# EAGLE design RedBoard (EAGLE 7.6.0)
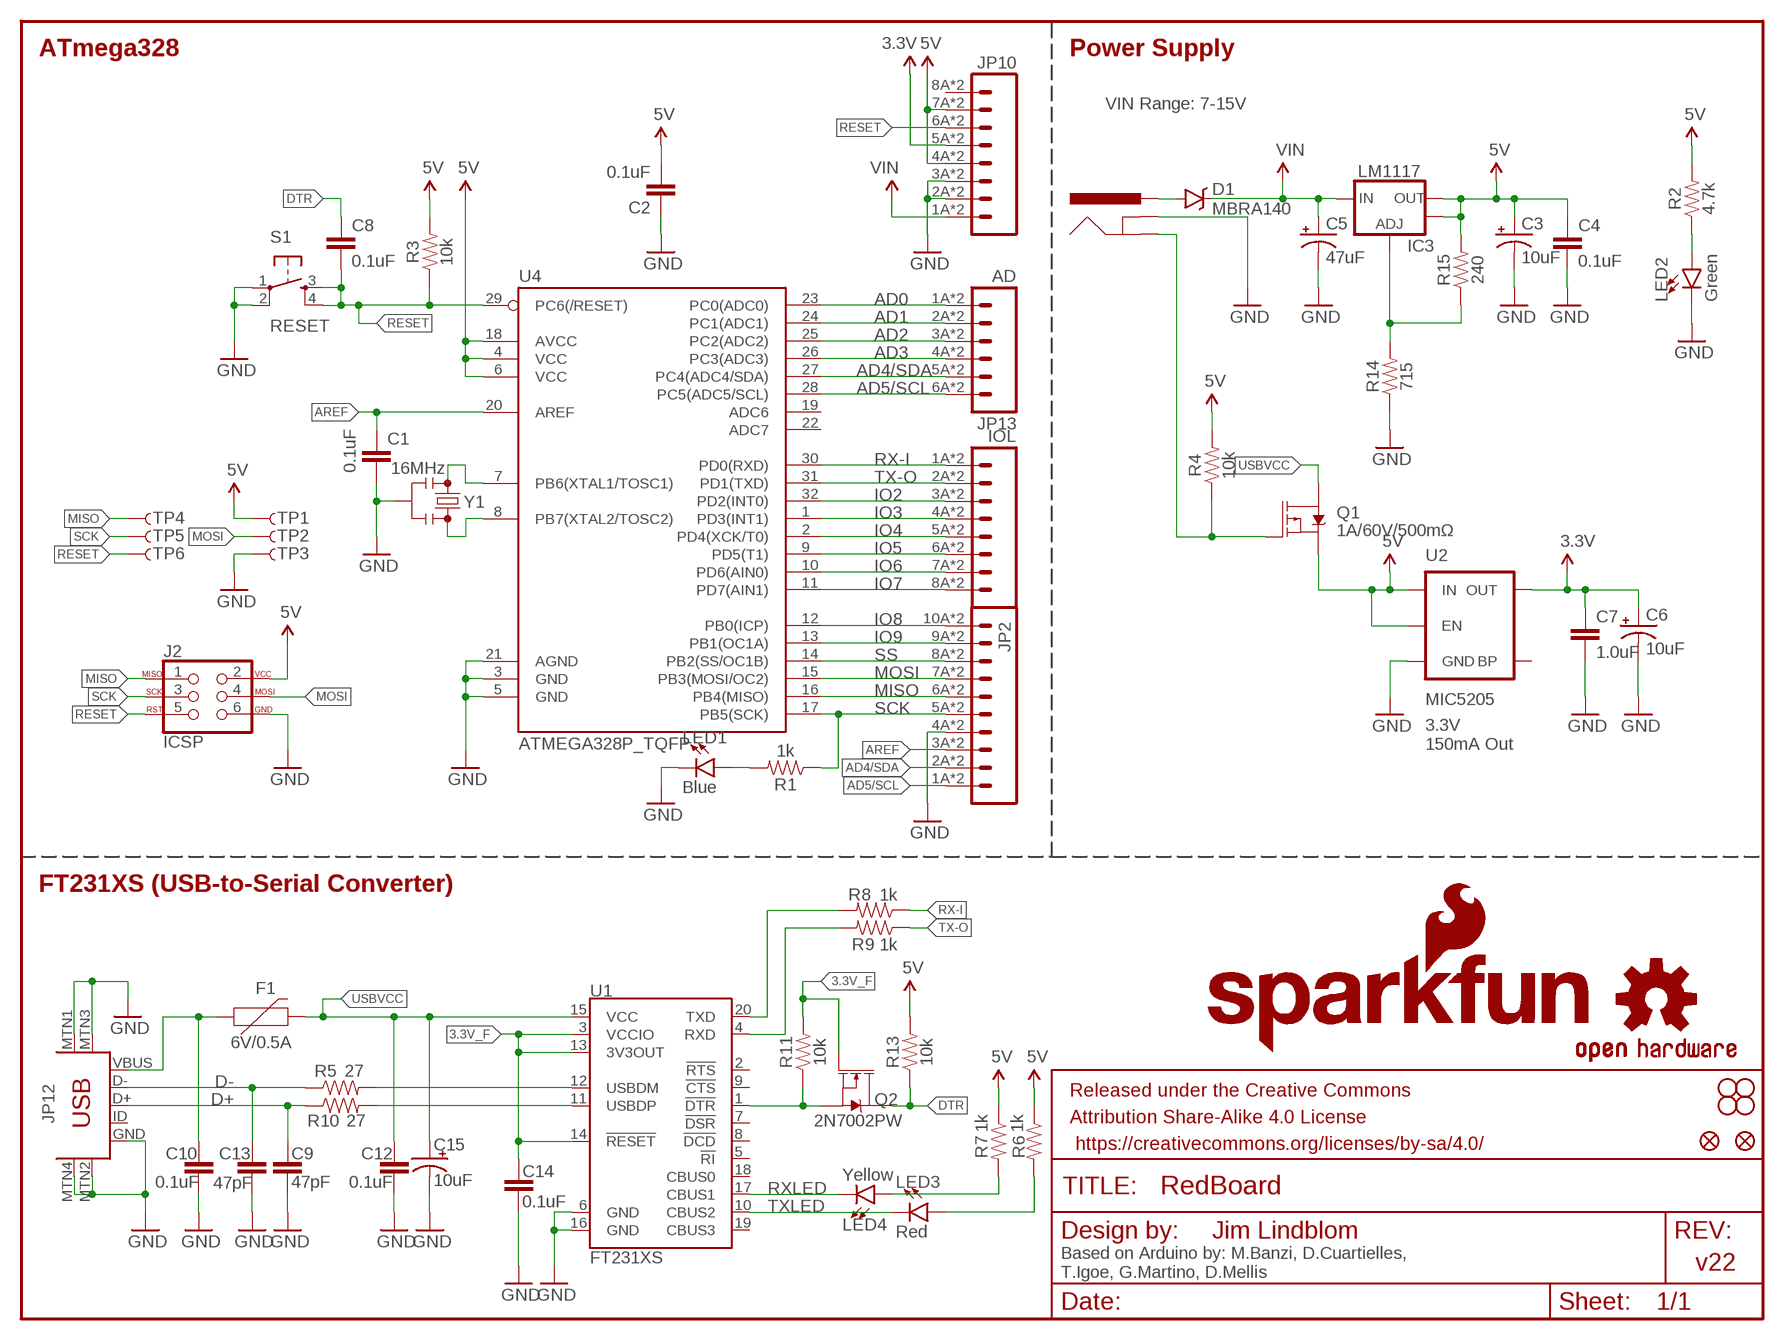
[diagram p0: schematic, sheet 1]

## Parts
C1  0.1uF  0.1UF-0603-25V-(+80/-20%)  [0603]
C2  0.1uF  0.1UF-0603-25V-(+80/-20%)  [0603]
C3  10uF  10UF-POLAR-EIA3216-16V-10%(TANT)  [EIA3216]
C4  0.1uF  0.1UF-0603-25V-(+80/-20%)  [0603]
C5  47uF  47UF-POLAR-PANASONIC_D-35V-20%  [PANASONIC_D]
C6  10uF  10UF-POLAR-EIA3216-16V-10%(TANT)  [EIA3216]
C7  1.0uF  1.0UF-0603-16V-10%  [0603]
C8  0.1uF  0.1UF-0603-25V-(+80/-20%)  [0603]
C9  47pF  47PF-0603-50V-5%  [0603]
C10  0.1uF  0.1UF-0603-25V-(+80/-20%)  [0603]
C12  0.1uF  0.1UF-0603-25V-(+80/-20%)  [0603]
C13  47pF  47PF-0603-50V-5%  [0603]
C14  0.1uF  0.1UF-0603-25V-(+80/-20%)  [0603]
C15  10uF  10UF-POLAR-EIA3216-16V-10%(TANT)  [EIA3216]
D1  MBRA140  [SMA-DIODE]
F1  6V/0.5A  PTC-HALF_AMP  [1206]
FRAME2  FRAME-LETTER  [CREATIVE_COMMONS]
IC3  LM1117  V_REG_LM1117ALT1  [SOT223-ALT1]
J2  ICSP  AVR_SPI_PROG_3X2SMD  [2X3_SMT_POSTS]
J3  POWER_JACKSUPER_BOMB_DIGITY  [POWER_JACK_SMD_OVERPASTE_SUPER_BOMB_DIGITY]
JP1  SFE_LOGO_NAME.1_INCH  [SFE_LOGO_NAME_.1]
JP2  M10SMD_COMBO  [1X10_SMD_COMBINED]
JP3  STAND-OFF  [STAND-OFF]
JP4  STAND-OFF  [STAND-OFF]
JP5  STAND-OFF  [STAND-OFF]
JP6  STAND-OFF  [STAND-OFF]
JP7  SFE_LOGO_FLAME.1_INCH  [SFE_LOGO_FLAME_.1]
JP8  FIDUCIAL1X2  [FIDUCIAL-1X2]
JP9  FIDUCIAL1X2  [FIDUCIAL-1X2]
JP10  M08SMD-COMBO  [1X08_SMD_COMBINED]
JP11  IOL  M08SMD-COMBO  [1X08_SMD_COMBINED]
JP12  USB-MINIB-5PIN  [USB-MINIB]
JP13  AD  M06SMD-STRAIGHT-COMBO  [1X06_SMD_STRAIGHT_COMBO]
LED1  Blue  LED1206  [LED-1206]
LED2  Green  LED1206  [LED-1206]
LED3  Red  LED1206  [LED-1206]
LED4  Yellow  LED1206  [LED-1206]
Q1  1A/60V/500mΩ  MOSFET-PCH-ZXMP6A13F  [SOT23-3]
Q2  2N7002PW  MOSFET-NCH-2N7002PW  [SOT323]
R1  1k  1KOHM-0603-1/10W-1%  [0603]
R2  4.7k  4.7KOHM-0603-1/10W-1%  [0603]
R3  10k  10KOHM-0603-1/10W-1%  [0603]
R4  10k  10KOHM-0603-1/10W-1%  [0603]
R5  27  27OHM-0603-1/10W-1%  [0603]
R6  1k  1KOHM-0603-1/10W-1%  [0603]
R7  1k  1KOHM-0603-1/10W-1%  [0603]
R8  1k  1KOHM-0603-1/10W-1%  [0603]
R9  1k  1KOHM-0603-1/10W-1%  [0603]
R10  27  27OHM-0603-1/10W-1%  [0603]
R11  10k  10KOHM-0603-1/10W-1%  [0603]
R13  10k  10KOHM-0603-1/10W-1%  [0603]
R14  715  715OHM-0603-1/10W-1%  [0603]
R15  240  240OHM-0603-1/10W-1%  [0603]
S1  RESET  SWITCH_SPST_4_PINSQUARE  [TACTILE-SWITCH-SMD]
TP1  TP-3x5  TEST-POINT3X5  [PAD.03X.05]
TP2  TP-3x5  TEST-POINT3X5  [PAD.03X.05]
TP3  TP-3x5  TEST-POINT3X5  [PAD.03X.05]
TP4  TP-3x5  TEST-POINT3X5  [PAD.03X.05]
TP5  TP-3x5  TEST-POINT3X5  [PAD.03X.05]
TP6  TP-3x5  TEST-POINT3X5  [PAD.03X.05]
U1  FT231XS  [SSOP20_L]
U2  MIC5205  MIC52053.3V  [SOT23-5]
U4  ATMEGA328P_TQFP  [TQFP32-08]
U$16  OSHW-LOGOS  [OSHW-LOGO-S]
Y1  16MHz  RESONATOR-16MHZSMD_3.2X1.3  [RESONATOR-SMD-3.2X1.3]

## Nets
3.3V: C6.+ C7.1 JP10.5A JP10.5B U2.5(OUT)
3.3V_F: C14.1 Q2.1(G) R11.2 U1.3(VCCIO) U1.13(3V3OUT) U1.14(!RESET)
5V: C2.2 C3.+ C4.1 IC3.2(OUT) IC3.4(OUT) J2.2 JP10.4A JP10.4B JP10.7A JP10.7B Q1.2(S) R2.2 R3.2 R4.2 R6.1 R7.1 R13.2 R15.2 TP1.P$1 U2.1(IN) U2.3(EN) U4.4(VCC) U4.6(VCC) U4.18(AVCC)
AD0: JP13.1A JP13.1B U4.23(PC0(ADC0))
AD1: JP13.2A JP13.2B U4.24(PC1(ADC1))
AD2: JP13.3A JP13.3B U4.25(PC2(ADC2))
AD3: JP13.4A JP13.4B U4.26(PC3(ADC3))
AD4/SDA: JP2.2A JP2.2B JP13.5A JP13.5B U4.27(PC4(ADC4/SDA))
AD5/SCL: JP2.1A JP2.1B JP13.6A JP13.6B U4.28(PC5(ADC5/SCL))
AREF: C1.1 JP2.3A JP2.3B U4.20(AREF)
D+: C9.1 JP12.D+ R10.1
D-: C13.1 JP12.D- R5.1
DTR: C8.1 Q2.3(D) R13.1
FTDI_DTR: Q2.2(S) R11.1 U1.1(!DTR)
GND: C1.2 C2.1 C3.- C4.2 C5.- C6.- C7.2 C9.2 C10.2 C12.2 C13.2 C14.2 C15.- J2.6 J3.GND(GNDBREAK) JP2.4A JP2.4B JP10.2A JP10.2B JP10.3A JP10.3B JP12.GND JP12.MTN1(MTN2) JP12.MTN2(MTN3) JP12.MTN3(MTN1) JP12.MTN4 LED1.C LED2.C R14.1 S1.1 S1.2 TP3.P$1 U1.6(GND) U1.16(GND) U2.2(GND) U4.3(GND) U4.5(GND) U4.21(AGND) Y1.2
INSERT: J3.P$4(GND) Q1.1(G) R4.1
IO2: JP11.3A JP11.3B U4.32(PD2(INT0))
IO3: JP11.4A JP11.4B U4.1(PD3(INT1))
IO4: JP11.5A JP11.5B U4.2(PD4(XCK/T0))
IO5: JP11.6A JP11.6B U4.9(PD5(T1))
IO6: JP11.7A JP11.7B U4.10(PD6(AIN0))
IO7: JP11.8A JP11.8B U4.11(PD7(AIN1))
IO8: JP2.10A JP2.10B U4.12(PB0(ICP))
IO9: JP2.9A JP2.9B U4.13(PB1(OC1A))
MISO: J2.1 JP2.6A JP2.6B TP4.P$1 U4.16(PB4(MISO))
MOSI: J2.4 JP2.7A JP2.7B TP2.P$1 U4.15(PB3(MOSI/OC2))
N$1: LED1.A R1.2
N$2: LED2.A R2.1
N$3: U4.7(PB6(XTAL1/TOSC1)) Y1.1
N$4: U4.8(PB7(XTAL2/TOSC2)) Y1.3
N$6: R5.2 U1.12(USBDM)
N$7: R10.2 U1.11(USBDP)
N$8: LED3.A R6.2
N$10: LED4.A R7.2
N$15: IC3.1(ADJ) R14.2 R15.1
PWRIN: D1.A J3.VIN0(PWR)
RESET: C8.2 J2.5 JP10.6A JP10.6B R3.1 S1.3 S1.4 TP6.P$1 U4.29(PC6(/RESET))
RX-I: JP11.1A JP11.1B R8.1 U4.30(PD0(RXD))
RXD: R9.2 U1.4(RXD)
RXLED: LED4.C U1.17(CBUS1)
SCK: J2.3 JP2.5A JP2.5B R1.1 TP5.P$1 U4.17(PB5(SCK))
SS: JP2.8A JP2.8B U4.14(PB2(SS/OC1B))
TX-O: JP11.2A JP11.2B R9.1 U4.31(PD1(TXD))
TXD: R8.2 U1.20(TXD)
TXLED: LED3.C U1.10(CBUS2)
USBVCC: C12.1 C15.+ F1.2 Q1.3(D) U1.15(VCC)
VIN: C5.+ D1.C IC3.3(IN) JP10.1A JP10.1B
VUSB: C10.1 F1.1 JP12.VBUS
Unconnected: JP10.8A JP10.8B JP12.ID U1.2(!RTS) U1.5(!RI) U1.7(!DSR) U1.8(!DCD) U1.9(!CTS) U1.18(CBUS0) U1.19(CBUS3) U2.4(BP) U4.19(ADC6) U4.22(ADC7)

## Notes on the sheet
- ATmega328 | Power Supply
- VIN Range: 7-15V
- 3.3V
  150mA Out
- FT231XS (USB-to-Serial Converter)
- Jim Lindblom
- v22
- Based on Arduino by: M.Banzi, D.Cuartielles, 
  T.Igoe, G.Martino, D.Mellis

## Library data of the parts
C1 C2 C4 C8 C10 C12 C14 = SparkFun-Capacitors:0.1UF: 0.1µF ceramic capacitors; PROD_ID: CAP-00810
C3 C6 C15 = SparkFun-Capacitors:10UF-POLAR: 10.0µF polarized capacitors; PROD_ID: CAP-00811
C5 = SparkFun-Capacitors:47UF-POLAR: 47µF polarized capacitors; PROD_ID: CAP-08478
C7 = SparkFun-Capacitors:1.0UF: 1µF ceramic capacitors; PROD_ID: CAP-00868
C9 C13 = SparkFun-Capacitors:47PF: 47pF ceramic capacitors; PROD_ID: CAP-08913
D1 = SparkFun-DiscreteSemi:MBRA140: 40V, 1A Schottky rectifier; PROD_ID: DIO-08053
F1 = SparkFun-Fuses:PTC: Resettable Fuse PTC; PROD_ID: RES-08585
FRAME2 = SparkFun-Aesthetics:FRAME-LETTER: Schematic Frame
IC3 = Testing:V_REG_LM1117: Voltage Regulator LM1117 Standard adjustable voltage regulator but in SMD form. Spark Fun Electronics SKU : COM-00595; PROD_ID: VREG-08170
J2 = SparkFun-Connectors:AVR_SPI_PROG_3X2: AVR ISP 6 Pin This is the reduced ISP connector for AVR programming. Common on Arduino. This footprint will take up less PCB space and can be used with a 10-pin to 6-pin adapter such as SKU: BOB-08508 **Special note about "TEST_POINT" package. The stop mask is on the top side, so if you want your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; PROD_ID: CONN-11415
J3 = Testing:POWER_JACK: Power Jack This is the standard 5.5mm barrel jack for power. The PTH is the most common, proven, reliable, footprint. All others are experimental. The Slot footprint only works if the mill layer is transmitted to the PCB fab house so be warned. Spark Fun Electronics SKU : PRT-00119. Mating wall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; PROD_ID: CONN-08106
JP1 = SparkFun-Aesthetics:SFE_LOGO_NAME: SFE Logo, name only
JP2 = SparkFun-Connectors:M10: Header 10 Standard 10-pin 0.1" header. Use with straight break away headers (SKU : PRT-00116), right angle break away headers (PRT-00553), swiss pins (PRT-00743), machine pins (PRT-00117), and female headers (PRT-00115).; PROD_ID: CONN-11219
JP3-JP6 = SparkFun:STAND-OFF: Stand Off
JP7 = SparkFun-Aesthetics:SFE_LOGO_FLAME: SFE Logo, flame only
JP8 JP9 = SparkFun:FIDUCIAL: Fiducial Alignment Points
JP10 JP11 = SparkFun-Connectors:M08: Header 8 Standard 8-pin 0.1" header. Use with straight break away headers (SKU : PRT-00116), right angle break away headers (PRT-00553), swiss pins (PRT-00743), machine pins (PRT-00117), and female headers (PRT-00115).; PROD_ID: CONN-10204
JP12 = SparkFun-Connectors:USB-MINIB: Mini-USB "B" connector with 5th pin broken out. Created new symbol breaking out 5th "ID" pin in mini/micro USB connector spec. See: http://en.wikipedia.org/wiki/Mini_usb#Cables. Uses same footprint as 4-pin symbol. Also added pins to connect to mounting / shield pads if required (probably not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; PROD_ID: CONN-08193
JP13 = SparkFun-Connectors:M06: Header 6 Standard 6-pin 0.1" header. Use with straight break away headers (SKU : PRT-00116), right angle break away headers (PRT-00553), swiss pins (PRT-00743), machine pins (PRT-00117), and female headers (PRT-00115). Molex polarized connector foot print use with SKU : PRT-08094 with associated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; PROD_ID: CONN-10203
LED1 = SparkFun-LED:LED: LED (Generic); PROD_ID: DIO-09911
LED2 = SparkFun-LED:LED: LED (Generic); PROD_ID: DIO-09910
LED3 = SparkFun-LED:LED: LED (Generic); PROD_ID: DIO-09912
LED4 = SparkFun-LED:LED: LED (Generic); PROD_ID: DIO-09909
Q1 = SparkFun-DiscreteSemi:MOSFET-PCH: P-channel MOSFETs Voltage controlled devices that allow control of high current outputs.; PROD_ID: TRANS-08285
Q2 = SparkFun-DiscreteSemi:MOSFET-NCH: N-channel MOSFETs Voltage controlled devices that allow control of high current outputs.; PROD_ID: TRANS-11151; VALUE: 310mA/60V/1.6Ω
R1 R6-R9 = SparkFun-Resistors:1KOHM: 1kΩ resistor; PROD_ID: RES-07856
R2 = SparkFun-Resistors:4.7KOHM: 4.7kΩ resistor; PROD_ID: RES-07857
R3 R4 R11 R13 = SparkFun-Resistors:10KOHM: 10kΩ resistor; PROD_ID: RES-00824
R5 R10 = SparkFun-Resistors:27OHM: 27Ω resistor; PROD_ID: RES-09334
R14 = SparkFun-Resistors:715OHM: 715Ω resistor; PROD_ID: RES-07850
R15 = SparkFun-Resistors:240OHM: 240Ω resistor; PROD_ID: RES-07849
S1 = SparkFun-Electromechanical:SWITCH_SPST_4_PIN; PROD_ID: SWCH-08247
TP1-TP4 TP6 = SparkFun-Connectors:TEST-POINT: Bare copper test points for troubleshooting or ICT
TP5 = SparkFun-Passives:TEST-POINT: Bare copper test points for troubleshooting or ICT
U1 = SparkFun-IC-Comms:FT231X: FTDI FT231X Full Speed USB to Full-handshake UART This USB2.0 Full Speed IC offers a compact bridge to full handshake UART interfaces. The device is a UART, capable of operating up to 3MBaud, with low power consumption (8mA). The FT231X includes the complete FT-X series feature set and enables USB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; PROD_ID: IC-11524
U2 = SparkFun-PowerIC:MIC5205: MIC5205 150mA vreg 3.3V - VREG-00822 5V - VREG-00823; PROD_ID: VREG-00822
U4 = SparkFun-IC-Microcontroller:ATMEGA328P_TQFP; PROD_ID: IC-09069
U$16 = SparkFun-Aesthetics:OSHW-LOGO: Open Source Hardware Logo
Y1 = SparkFun-Clocks:RESONATOR-16MHZ: 16MHz Resonator Digikey Example Frequency: 16MHz Frequency Stability: &plusmn;0.3% Frequency Tolerance: &plusmn;0.5% Capacitance: 15pF; PROD_ID: XTAL-08900

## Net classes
0 default: width 0.152 mm, drill 0.305 mm, clearance 0.152 mm

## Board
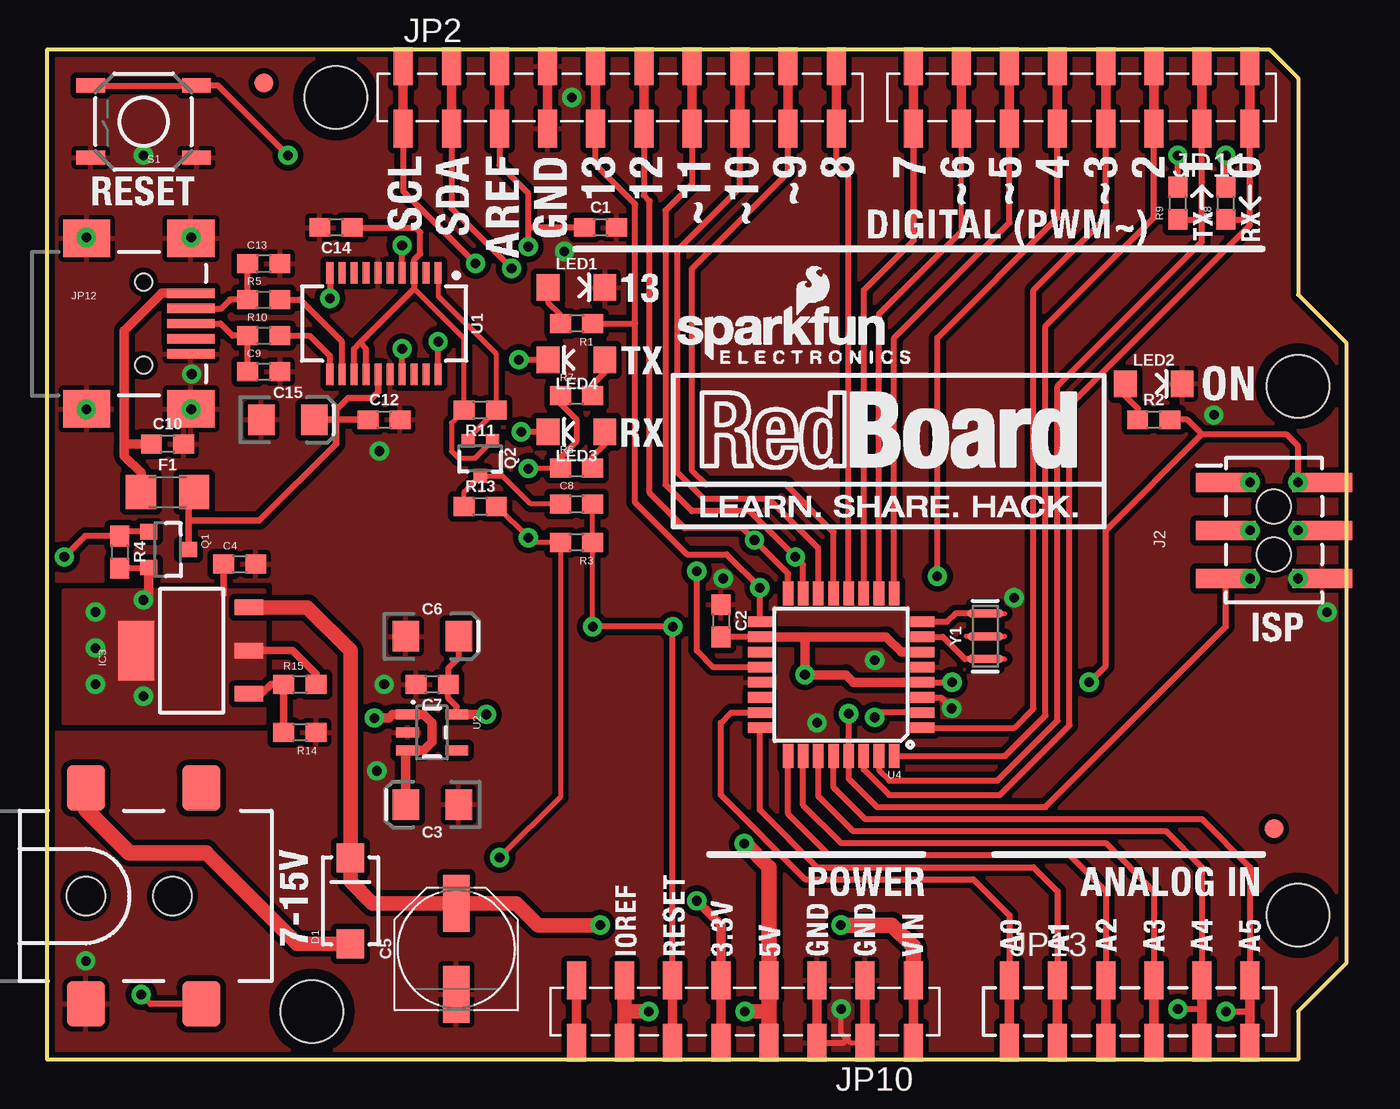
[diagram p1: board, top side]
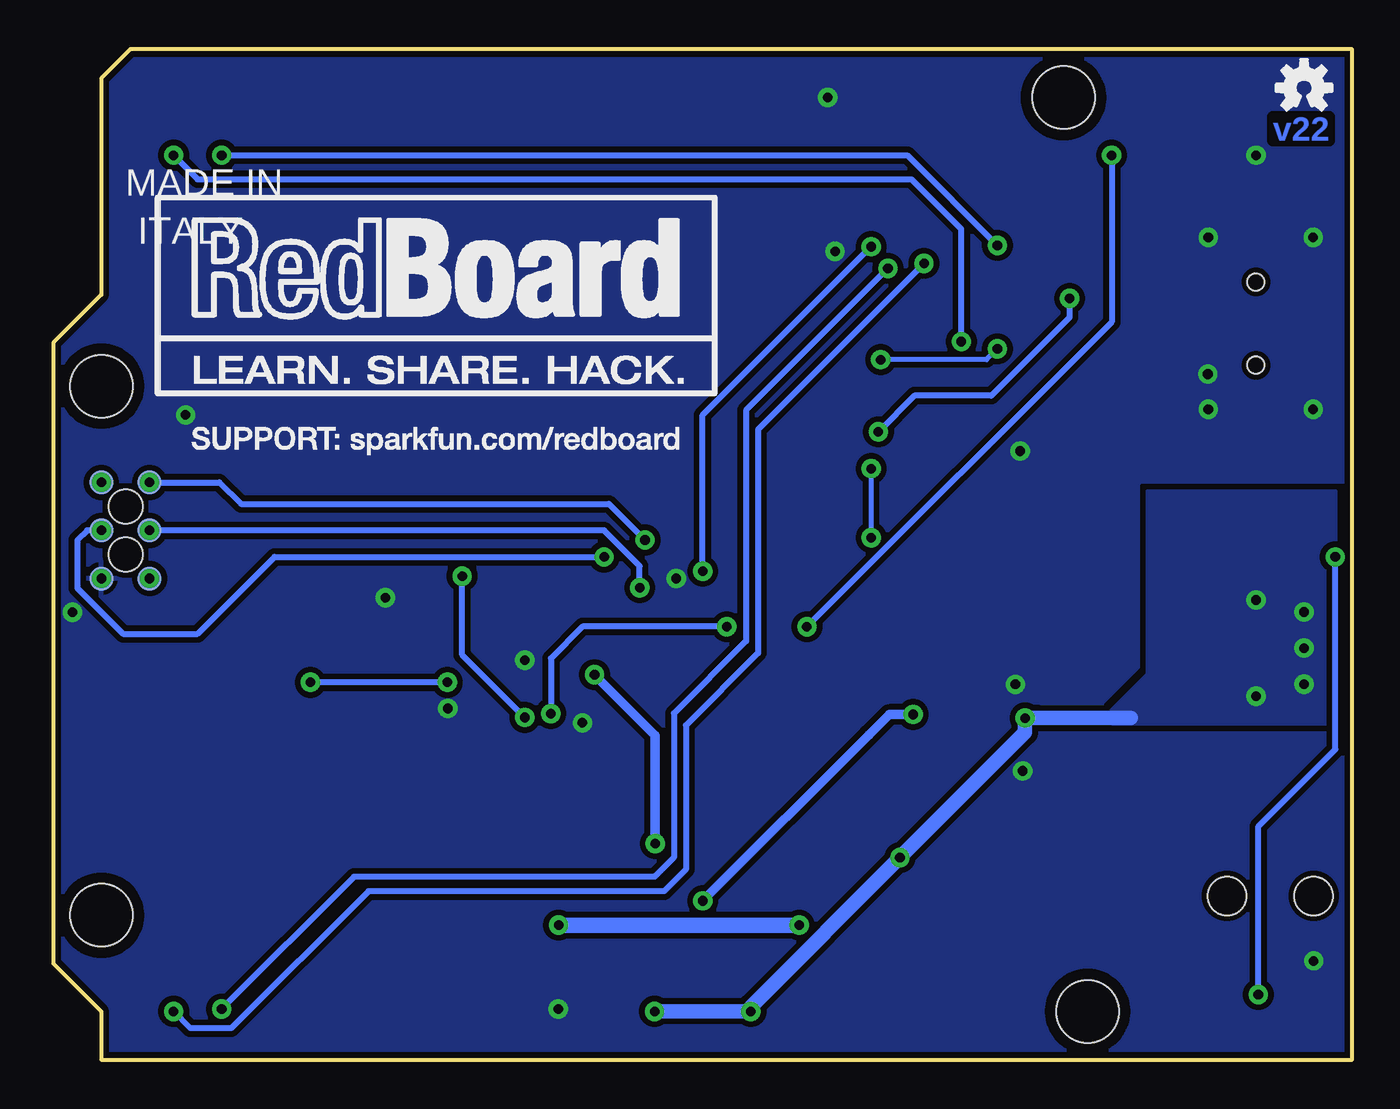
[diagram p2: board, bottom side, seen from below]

Size 68.58 x 53.34 mm. Coordinates in mm from the lower left corner, seen from the top.
Outline: 0,53.34 64.52,53.34 66.04,51.82 66.04,40.39 68.58,37.85 68.58,5.08 66.04,2.54 66.04,0 0,0 0,53.34
Copper layers (1*16): Top 0.035mm / dielectric 1.5mm / Bottom 0.035mm
Design rules "SparkFun-2-layer": minimum track width 7mil, minimum drill 15mil, track to track 8mil, track to pad 8mil, pad to pad 8mil, via to via 8mil, smd to smd 8mil, copper to edge 8mil, drill to drill 8mil, minimum pad ring 12mil, minimum via ring 10mil, stop-mask expansion 4mil, vias tented up to drill 20mil, thermal gap 10mil
vRestrict: area 0.6,22.4 to 2,30.6; area 5.7,23.1 to 7.4,30.6; area 47.9,10.8 to 48.5,11.3; area 50.4,10.7 to 50.9,11.6; area 11.3,29.3 to 12.7,31.6; area 0.3,13 to 9.4,25

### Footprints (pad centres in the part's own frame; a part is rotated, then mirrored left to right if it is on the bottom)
0603 = smd 1.1 x 1: 1 -0.85,0; 2 0.85,0
EIA3216 = smd 1.4 x 1.6: + 1.4,0; - -1.4,0
PANASONIC_D = smd 3 x 1.4: + 2.4,0; - -2.4,0
SMA-DIODE = smd 1.524 x 1.47: A -2.277,0; C 2.277,0
1206 = smd 1.6 x 1.8: 1 -1.4,0; 2 1.4,0
SOT223-ALT1 = smd 0.813 x 1.524: 1 -2.271,-3.02; 2 0,-3.02; 3 2.288,-3.02 | smd 3.124 x 1.905: 4 0,2.921
2X3_SMT_POSTS = smd 1 x 3.17: 1 -2.54,-2.54; 2 -2.54,2.54; 3 0,-2.54; 4 0,2.54; 5 2.54,-2.54; 6 2.54,2.54 | hole 1.8: -1.27,0; 1.27,0
POWER_JACK_SMD_OVERPASTE_SUPER_BOMB_DIGITY = smd 2 x 2.4: GND 0,-5.7; P$4 6.1,-5.7; VIN0 0,5.7; VIN1 6.1,5.7 | hole 2.032: 0,0; 4.572,0
1X10_SMD_COMBINED = smd 1 x 2: 1A 0,1.65; 1B 0,-1.65; 2A 2.54,1.65; 2B 2.54,-1.65; 3A 5.08,1.65; 3B 5.08,-1.65; 4A 7.62,1.65; 4B 7.62,-1.65; 5A 10.16,1.65; 5B 10.16,-1.65; 6A 12.7,1.65; 6B 12.7,-1.65; 7A 15.24,1.65; 7B 15.24,-1.65; 8A 17.78,1.65; 8B 17.78,-1.65; 9A 20.32,1.65; 9B 20.32,-1.65; 10A 22.86,1.65; 10B 22.86,-1.65
STAND-OFF = hole 3.302: 0,0
FIDUCIAL-1X2 = smd 1 x 1: 1 0,0
1X08_SMD_COMBINED = smd 1 x 2: 1A 0,1.65; 1B 0,-1.65; 2A 2.54,-1.65; 2B 2.54,1.65; 3A 5.08,1.65; 3B 5.08,-1.65; 4A 7.62,-1.65; 4B 7.62,1.65; 5A 10.16,1.65; 5B 10.16,-1.65; 6A 12.7,-1.65; 6B 12.7,1.65; 7A 15.24,1.65; 7B 15.24,-1.65; 8A 17.78,-1.65; 8B 17.78,1.65
USB-MINIB = smd 2.5 x 0.5: D+ 2.5,0; D- 2.5,0.8; GND 2.5,-1.6; ID 2.5,-0.8; VBUS 2.5,1.6 | smd 2.5 x 2: MTN1 -3,4.5; MTN2 2.5,4.5; MTN3 -3,-4.5; MTN4 2.5,-4.5 | hole 0.9: 0,2.2; 0,-2.2
1X06_SMD_STRAIGHT_COMBO = smd 1 x 2: 1A 0,-1.65; 1B 0,1.65; 2A 2.54,1.65; 2B 2.54,-1.65; 3A 5.08,-1.65; 3B 5.08,1.65; 4A 7.62,1.65; 4B 7.62,-1.65; 5A 10.16,-1.65; 5B 10.16,1.65; 6A 12.7,1.65; 6B 12.7,-1.65
LED-1206 = smd 1.2 x 1.4: A -1.5,0; C 1.5,0
SOT23-3 = smd 0.8 x 0.9: 1 -0.95,-1; 2 0.95,-1; 3 0,1.1
SOT323 = smd 0.7 x 0.7: 1 -0.65,-0.925; 2 0.65,-0.925; 3 0,0.925
TACTILE-SWITCH-SMD = smd 1.524 x 0.762: 1 -2.794,1.905; 2 2.794,1.905; 3 -2.794,-1.905; 4 2.794,-1.905
PAD.03X.05 = smd 1.27 x 1.27: P$1 0,0
SSOP20_L = smd 0.381 x 1.143: 1 -2.857,-2.68; 2 -2.223,-2.68; 3 -1.587,-2.68; 4 -0.953,-2.68; 5 -0.318,-2.68; 6 0.318,-2.68; 7 0.953,-2.68; 8 1.587,-2.68; 9 2.223,-2.68; 10 2.857,-2.68; 11 2.857,2.68; 12 2.223,2.68; 13 1.587,2.68; 14 0.953,2.68; 15 0.318,2.68; 16 -0.318,2.68; 17 -0.953,2.68; 18 -1.587,2.68; 19 -2.223,2.68; 20 -2.857,2.68
SOT23-5 = smd 0.55 x 1.2: 1 -0.95,-1.3; 2 0,-1.3; 3 0.95,-1.3; 4 0.95,1.3; 5 -0.95,1.3
TQFP32-08 = smd 1.27 x 0.559: 1 -4.293,2.8; 2 -4.293,2; 3 -4.293,1.2; 4 -4.293,0.4; 5 -4.293,-0.4; 6 -4.293,-1.2; 7 -4.293,-2; 8 -4.293,-2.8; 17 4.293,-2.8; 18 4.293,-2; 19 4.293,-1.2; 20 4.293,-0.4; 21 4.293,0.4; 22 4.293,1.2; 23 4.293,2; 24 4.293,2.8 | smd 0.559 x 1.27: 9 -2.8,-4.293; 10 -2,-4.293; 11 -1.2,-4.293; 12 -0.4,-4.293; 13 0.4,-4.293; 14 1.2,-4.293; 15 2,-4.293; 16 2.8,-4.293; 25 2.8,4.293; 26 2,4.293; 27 1.2,4.293; 28 0.4,4.293; 29 -0.4,4.293; 30 -1.2,4.293; 31 -2,4.293; 32 -2.8,4.293
RESONATOR-SMD-3.2X1.3 = smd 0.45 x 1.905: 1 -1.2,0; 2 0,0; 3 1.2,0

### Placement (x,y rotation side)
C1  29.21,43.94 0 top
C2  35.56,23.17 270 top
C3  20.32,13.46 180 top
C4  10.16,26.16 0 top
C5  21.59,5.84 90 top
C6  20.32,22.35 0 top
C7  20.32,19.81 180 top
C8  27.94,29.34 0 top
C9  11.43,36.32 0 top
C10  6.35,32.51 0 top
C12  17.78,33.78 0 top
C13  11.43,42.04 0 top
C14  15.24,43.94 180 top
C15  12.7,33.78 0 top
D1  16,8.38 90 top
F1  6.35,29.97 0 top
FRAME2  not placed on the board
IC3  7.62,21.59 90 top
J2  64.77,27.94 270 top
J3  2.03,8.64 0 top
JP1  32.79,36.45 0 top
JP2  18.8,50.8 0 top
JP3  13.97,2.54 0 top
JP4  66.04,7.62 0 top
JP5  66.04,35.56 0 top
JP6  15.24,50.8 0 top
JP7  39.27,38.99 0 top
JP8  64.77,12.19 0 top
JP9  11.43,51.56 0 top
JP10  45.72,2.54 180 top
JP11  63.5,50.8 180 top
JP12  5.08,38.86 0 top
JP13  50.8,2.54 0 top
LED1  27.94,40.77 0 top
LED2  58.42,35.69 0 top
LED3  27.94,33.15 180 top
LED4  27.94,36.96 180 top
Q1  6.35,26.92 270 top
Q2  22.86,31.75 180 top
R1  27.94,38.86 180 top
R2  58.42,33.78 0 top
R3  27.94,27.3 180 top
R4  3.81,26.8 270 top
R5  11.43,40.13 0 top
R6  27.94,31.24 0 top
R7  27.94,35.05 0 top
R8  62.23,45.21 90 top
R9  59.69,45.21 90 top
R10  11.43,38.23 0 top
R11  22.86,34.29 180 top
R13  22.86,29.21 0 top
R14  13.34,17.27 180 top
R15  13.34,19.81 0 top
S1  5.08,49.53 180 top
TP1  66.04,30.48 0 bottom
TP2  66.04,27.94 0 bottom
TP3  66.04,25.4 0 bottom
TP4  63.5,30.48 0 bottom
TP5  63.5,27.94 0 bottom
TP6  63.5,25.4 0 bottom
U1  17.78,38.86 180 top
U2  20.32,17.27 270 top
U4  41.91,20.32 180 top
U$16  2.54,51.31 0 bottom
Y1  49.53,22.35 90 top

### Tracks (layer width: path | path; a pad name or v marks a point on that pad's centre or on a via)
3.3V  (via drill 0.51)
  Top 0.305: U2.5 21.62,18.64 21.17,19.09 C7.1 21.17,20.66 21.72,21.21 C6.+
  Top 0.508: JP10.5A 35.56,7.11 v34.29,8.38 | U2.5 v23.18,18.22
  Bottom 0.508: v34.29,8.38 25.53,17.14 25.52,17.14 24.45,18.22 v23.18,18.22
3.3V_F
  Top 0.254: 19.37,40.7 22.01,38.06 R11.2 21.34,33.62 21.34,32.13 21.72,31.75 22.59,31.75 Q2.1
  Top 0.305: C14.1 19.43,43.94 19.68,43.69 19.68,42.55 19.37,42.23 U1.3 19.37,40.7 16.51,37.85 | U1.13 16.19,37.53 16.51,37.85 | U1.14 16.83,37.53 16.51,37.85
5V  (via drill 0.51, 0.51 pad 0.51)
  Top 0.254: 27.09,31.2 v25.4,31.2 | R13.2 23.75,29.21 v25.4,27.56 25.65,27.3 R3.2 27.09,13.88 v23.88,10.67
  Top 0.305: U4.18 C2.2 | U4.4 v47.77,19.92 | 60.96,33.02 65.41,33.02 66.04,32.38 TP1.P$1 J2.2 | JP10.4A 38.1,2.03 | 60.96,33.02 55.88,27.94 55.88,20.79 v55.01,19.92 | 60.96,33.02 60.2,33.78 R2.2 | R7.1 27.09,34.63 27.94,33.78 27.94,32.64 27.09,31.79 R6.1 27.09,31.2 | R4.2 5.32,25.95 Q1.2
  Top 0.356: C4.1 9.31,24.55
  Top 0.406: IC3.2 12.95,21.59 14.19,20.36 R15.2 | C3.+ 19.05,13.46
  Top 0.508: U4.6 45.09,21.52 44.28,22.32 40.01,22.32 | 40.01,22.32 U4.18 | 40.01,22.32 v40.01,20.32 42.16,20.32 42.56,19.92 U4.4 | C3.+ 18.92,16.22 U2.3 19.88,16.32 20.32,16.76 20.32,17.78 19.88,18.22 U2.1 18.22,18.22 18.03,18.03 v17.27,18.03 | Q1.2 5.35,24.54 v5.08,24.27
  Top 0.762: v36.8,11.4 36.8,11.46 38.1,10.16 | v36.83,2.54 37.85,2.54 38.1,2.79 | v31.75,2.54 30.48,2.54 | 30.48,2.54 JP10.7A | JP10.7B 30.48,2.54
  Top 0.813: 38.1,10.16 JP10.4A 38.1,2.79 38.1,2.03 JP10.4B
  Bottom 0.254: v25.4,31.2 v25.4,27.56
  Bottom 0.305: v47.77,19.92 v55.01,19.92
  Bottom 0.508: v36.8,11.4 36.8,17.11 v40.01,20.32
  Bottom 0.762: v36.83,2.54 v31.75,2.54 31.75,2.79 v23.88,10.67 17.27,17.27 v17.27,18.03 | v17.27,18.03 11.68,18.03 | 16.51,18.03 v17.27,18.03
  other vias: 2.54,21.73 5.08,19.19 2.54,19.82 2.54,23.63 66.04,30.48
  pour Bottom (isolate 0.305, no thermals): 0.89,29.97 10.79,29.97 10.79,20.32 12.7,18.41 12.7,17.78 0.89,17.78
  pour Top (isolate 0.305, no thermals): 0.89,17.78 0.89,24.77 11.43,24.77 11.43,17.78
AD0
  Top 0.305: U4.23 36.1,18.32 35.56,17.78 35.56,13.97 40.01,9.53 48.9,9.53 50.8,7.62 JP13.1A
AD1
  Top 0.305: U4.24 37.62,13.18 40.64,10.16 52.07,10.16 53.34,8.89 JP13.2A
AD2
  Top 0.305: U4.25 39.11,12.96 41.27,10.79 53.98,10.79 55.88,8.89 JP13.3A
AD3
  Top 0.305: U4.26 39.91,13.43 41.91,11.43 55.88,11.43 58.42,8.89 JP13.4A
AD4/SDA  (via drill 0.51)
  Top 0.305: U4.27 40.71,13.9 42.55,12.06 59.05,12.06 60.96,10.16 60.96,2.67 | 60.96,2.67 JP13.5A | JP2.2B 21.34,44.96 v24.51,41.78 | v59.69,2.67 60.96,2.67
  Bottom 0.305: v59.69,2.67 52.7,9.65 36.83,9.65 35.81,10.67 35.81,18.29 32,22.1 32,34.29 v24.51,41.78
AD5/SCL  (via drill 0.51)
  Top 0.305: U4.28 41.51,14.37 43.18,12.7 60.96,12.7 63.5,10.16 JP13.6A 63.5,2.54 v62.23,2.54 | JP2.1B 18.8,45.85 v22.61,42.04
  Bottom 0.305: v22.61,42.04 31.37,33.27 31.37,21.46 35.18,17.65 35.18,10.03 36.32,8.89 51.94,8.89 59.18,1.65 61.34,1.65 v62.23,2.54
AREF  (via drill 0.51)
  Top 0.305: U4.20 35.16,20.72 34.29,21.59 v34.29,25.78 | JP2.3B 23.88,47.24 25.4,45.72 25.4,43.94 | v25.4,42.93 25.4,43.94 | C1.1 25.4,43.94
  Bottom 0.305: v25.4,42.93 34.29,34.04 v34.29,25.78
D+
  Top 0.305: R10.1 10.58,38.44 | JP12.D+ 9.14,38.86 9.78,38.23 R10.1 | C9.1 R10.1
D-
  Top 0.305: JP12.D- 9.18,39.66 9.65,40.13 R5.1 C13.1
DTR
  Top 0.254: R13.1 22.01,29.98 Q2.3 24.04,30.82 25.53,29.34 C8.1
FTDI_DTR
  Top 0.254: U1.1 20.64,40.32 23.71,37.25 R11.1 22.21,32.79 Q2.2
GND  (via drill 0.51, 0.51 pad 0.51)
  Top 0.254: JP10.2B 42.42,0.89 42.23,1.08 41.91,1.4 v41.91,2.67
  Top 0.305: U4.3 47.17,19.12 v47.75,18.54 | JP10.3A 42.04,0.89 42.23,1.08
  other vias: 5.08,47.75 61.59,34.04 40.64,17.78 27.69,50.8 43.69,21.08 51.05,24.38 35.69,25.4 2.03,5.21 7.62,36.2 27.3,42.67 67.56,23.62 17.53,32.13 17.78,19.81 17.4,15.24 66.04,25.4 2.06,34.34 7.59,34.34 2.06,43.41 7.59,43.41
  pour Top (isolate 0.305, rank 2): 0,53.34 64.52,53.34 66.04,51.82 66.04,40.39 68.58,37.85 68.58,5.08 66.04,2.54 66.04,0 0,0
  pour Bottom (isolate 0.305, rank 2): 0,53.34 64.52,53.34 66.04,51.82 66.04,40.39 68.58,37.85 68.58,5.08 66.04,2.54 66.04,0 0,0
INSERT  (via drill 0.51)
  Top 0.305: J3.P$4 5.45,2.94 v4.95,3.43 | Q1.1 4.04,27.87 R4.1 1.99,27.65 v0.89,26.54
  Bottom 0.305: v4.95,3.43 4.95,12.32 0.89,16.38 v0.89,26.54
IO2
  Top 0.305: JP11.3A 58.42,44.45 52.7,38.73 52.7,18.16 50.57,16.03 U4.32
IO3
  Top 0.305: JP11.4A 55.88,44.45 52.07,40.64 52.07,18.54 51.05,17.52 U4.1
IO4  (via drill 0.51)
  Top 0.305: v46.99,25.53 46.99,38.1 53.34,44.45 JP11.5A | U4.2 43.94,18.32 v43.69,18.07
  Bottom 0.305: v43.69,18.07 46.99,21.37 v46.99,25.53
IO5
  Top 0.305: U4.9 44.71,38.1 50.8,44.19 JP11.6A
IO6
  Top 0.254: 48.26,43.72 JP11.7A
  Top 0.305: U4.10 43.91,39.37 48.26,43.72
IO7
  Top 0.305: U4.11 43.11,40.64 45.72,43.25
  Top 0.356: 45.72,43.25 JP11.8A
IO8
  Top 0.305: U4.12 42.31,46.59 41.66,47.24 JP2.10B
IO9
  Top 0.305: JP2.9B 39.12,46.84 34.04,41.76 34.04,31.11 34.8,30.35 38.99,30.35 41.51,27.83 U4.13
MISO  (via drill 0.51, 0.51 pad 0.51)
  Top 0.305: U4.16 39.11,25.66 v37.34,27.43 36.7,28.07 33.66,28.07 31.8,29.92 31.8,45.34 31.5,45.64 JP2.6B | J2.1 TP4.P$1
  Bottom 0.305: v37.34,27.43 39.24,29.34 58.67,29.34 59.82,30.48 TP4.P$1
  other vias: 63.5,30.48
MOSI  (via drill 0.51, 0.51 pad 0.51)
  Top 0.305: U4.15 39.91,26.13 v39.5,26.54 37.08,28.96 34.04,28.96 32.64,30.35 32.64,44.83 34.04,46.23 JP2.7B | J2.4 TP2.P$1
  Bottom 0.305: v39.5,26.54 56.9,26.54 60.96,22.48 64.9,22.48 67.31,24.89 67.31,27.43 66.8,27.94 TP2.P$1
  other vias: 66.04,27.94
N$1
  Top 0.305: R1.2 27.09,39.33 26.44,39.98 LED1.A
N$2
  Top 0.356: R2.1 57.57,34.38 56.92,35.03 LED2.A
N$3
  Top 0.305: U4.7 47.28,22.32 48.44,21.15 Y1.1
N$4
  Top 0.305: U4.8 47.5,23.12 47.94,23.55 Y1.3
N$6
  Top 0.305: R5.2 13.34,40.13 15.56,37.91 U1.12
N$7
  Top 0.305: U1.11 14.92,37.15 13.84,38.23 R10.2
N$8
  Top 0.305: LED3.A 29.44,32.49 28.79,31.84 R6.2
N$10
  Top 0.305: LED4.A 29.44,36.3 28.79,35.65 R7.2
N$15
  Top 0.406: IC3.1 11.32,19.32 11.81,19.81 R15.1 R14.2
PWRIN
  Top 0.762: 8.38,10.92 13.2,6.11 D1.A
  Top 0.813: 8.38,10.92 4.32,10.92 2.03,13.21 J3.VIN0
RESET  (via drill 0.51, 0.51 pad 0.51)
  Top 0.254: C8.2 R3.1 v28.79,22.86
  Top 0.305: v42.31,18.27 U4.29 42.31,14.84 43.81,13.34 52.7,13.34 62.23,22.86 J2.5 TP6.P$1 | v12.7,47.75 9.02,51.44 S1.3 S1.4 | JP10.6B JP10.6A v33.02,22.86 v28.79,22.86
  Bottom 0.305: v42.31,18.27 42.31,21.19 40.64,22.86 v33.02,22.86 | v12.7,47.75 12.7,38.95 v28.79,22.86
  other vias: 63.5,25.4
RX-I
  Top 0.254: 63.5,46.35 63.52,46.37
  Top 0.305: 63.5,44.32 63.5,44.07 53.98,34.54 53.98,17.65 50.29,13.97 44.45,13.97 43.11,15.31 U4.30 | 63.5,44.32 63.5,46.35 JP11.1A | R8.1 63.46,44.36 63.5,44.32
RXD  (via drill 0.51)
  Top 0.305: R9.2 v59.69,47.75 | U1.4 v18.73,42.99
  Bottom 0.305: v59.69,47.75 23.5,47.75 v18.73,42.99
RXLED  (via drill 0.51)
  Top 0.305: U1.17 v18.73,37.53 | v24.89,36.96 LED4.C
  Bottom 0.254: v18.73,37.53 19.3,36.96 v24.89,36.96
SCK  (via drill 0.51, 0.51 pad 0.51)
  Top 0.305: U4.17 v37.62,24.92 35.87,26.67 33.78,26.67 31.04,29.41 31.04,38.86 | JP2.5B 28.96,47.24 31.04,45.16 31.04,38.86 | R1.1 31.04,38.86 | J2.3 TP5.P$1
  Bottom 0.305: v37.62,24.92 37.62,26.06 39.5,27.94 TP5.P$1
  other vias: 63.5,27.94
SS
  Top 0.305: JP2.8B 36.58,46.04 33.27,42.74 33.27,30.99 34.67,29.59 38.1,29.59 40.71,26.98 U4.14
TX-O
  Top 0.254: 60.96,46.35 60.95,46.37
  Top 0.305: U4.31 43.91,15.27 44.45,14.73 50.16,14.73 53.34,17.91 53.34,35.56 60.96,43.18 60.96,44.32 | 60.96,44.32 60.96,46.35 JP11.2A | R9.1 60.92,44.36 60.96,44.32
TXD  (via drill 0.51)
  Top 0.305: R8.2 v62.23,47.75 | U1.20 v20.64,37.91
  Bottom 0.305: v62.23,47.75 60.96,46.48 23.27,46.48 20.64,43.85 v20.64,37.91
TXLED  (via drill 0.51)
  Top 0.305: U1.10 v14.92,40.2 | LED3.C v25.02,33.15
  Bottom 0.305: v14.92,40.2 14.92,39.18 19.05,35.05 23.11,35.05 v25.02,33.15
USBVCC
  Top 0.356: C15.+ 15.24,33.78 | U1.15 17.46,35.24 17.14,34.92 15.88,34.92 15.24,34.29 15.24,33.78 | C12.1 15.24,33.78 | 15.24,33.78 15.24,32.51 11.18,28.45 7.45,28.45 | Q1.3 7.45,28.45 | 7.45,28.45 7.45,29.68 F1.2
VIN  (via drill 0.51)
  Top 0.305: JP10.1A JP10.1B
  Top 0.762: v29.2,7.1 25.9,7.1 24.76,8.24 C5.+ 17.16,8.24 16,9.4 D1.C 16,21.59 13.72,23.88 IC3.3
  Top 0.813: v41.9,7.1 44.59,7.1 45.72,5.97 JP10.1B
  Bottom 0.813: v29.2,7.1 v41.9,7.1
VUSB
  Top 0.508: 4.06,32.51 4.06,38.48 6.04,40.46 JP12.VBUS | C10.1 4.06,32.51 | 4.06,32.51 4.06,31.88 4.95,30.99 F1.1

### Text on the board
Bottom: v22
bNames: MADE IN | ITALY
Measures: Units in inches
tDocu: J.Lindblom | Based on Arduino by: M.Banzi, D.Cuartielles, / T.Igoe, G.Martino, D.Mellis
214bmp: D:/SmartProjects/Snc/a4_bn_logo2.bmp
